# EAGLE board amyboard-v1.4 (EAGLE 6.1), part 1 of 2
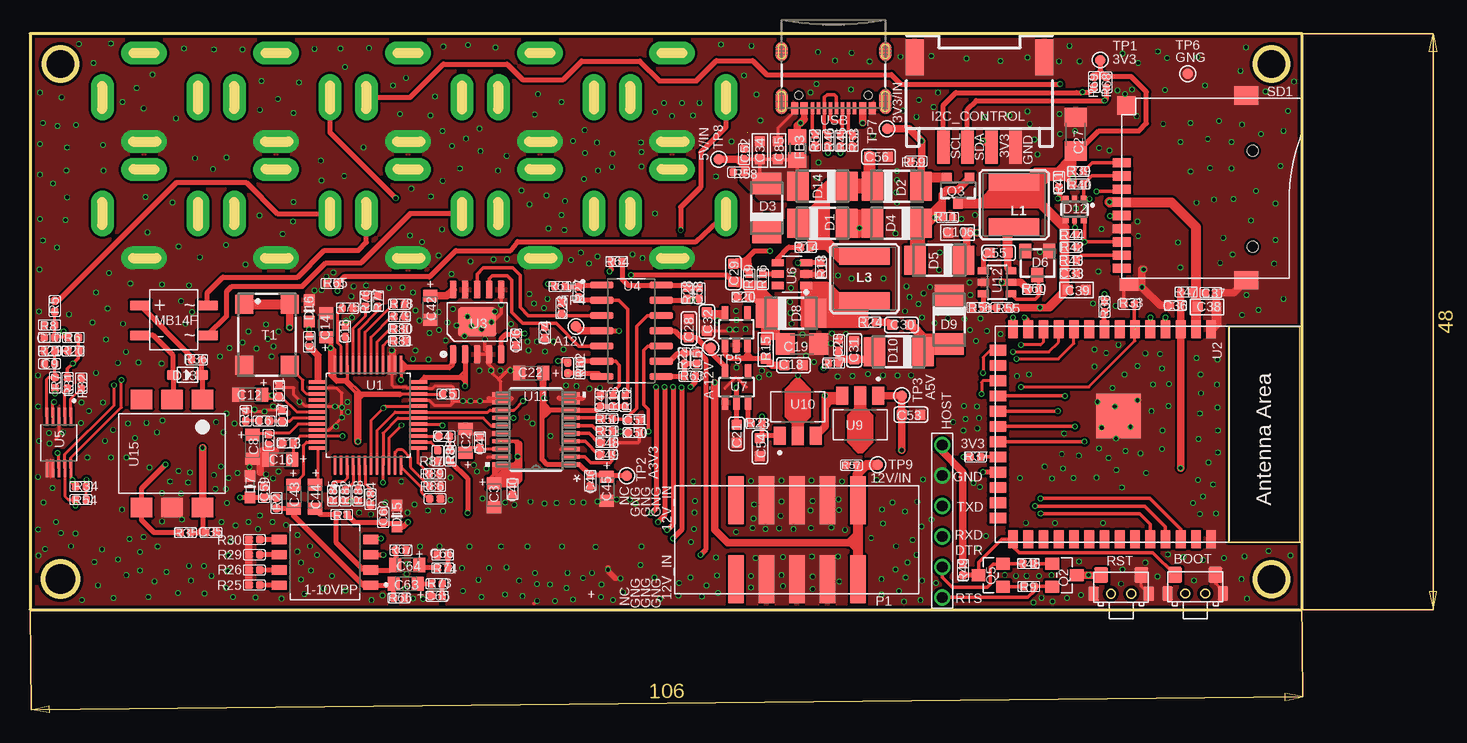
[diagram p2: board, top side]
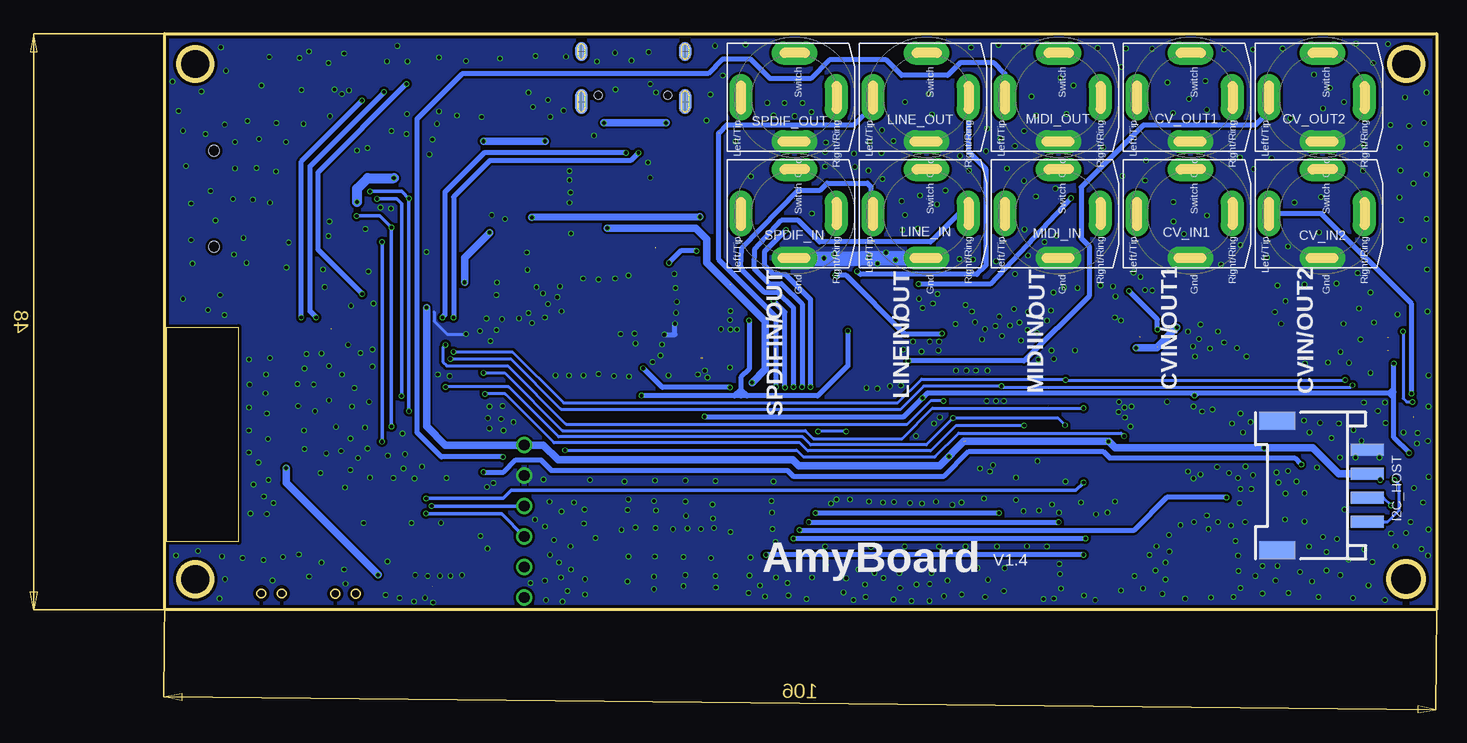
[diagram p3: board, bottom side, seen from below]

Size 117.22 x 56.61 mm. Coordinates in mm from the lower left corner, seen from the top.
Outline: 0,8.61 106,8.61 106,56.61 0,56.61 0,8.61
Outline: circle at 2.54,54.08 radius 1.37
Outline: circle at 2.54,11.15 radius 1.44
Outline: circle at 103.45,11.15 radius 1.37
Outline: circle at 103.45,54.08 radius 1.37
Copper layers (1*16): Top 0.035mm / dielectric 1.5mm / Bottom 0.035mm
Design rules: minimum track width 6mil, minimum drill 0.3mm, track to track 6mil, track to pad 6mil, pad to pad 6mil, via to via 6mil, smd to smd 0mil, copper to edge 10mil, drill to drill 8mil, minimum pad ring 3mil, minimum via ring 3mil, stop-mask expansion 0mil, vias tented up to drill 100mil, thermal gap 0mil
Net classes: 0 default: width 0.203 mm

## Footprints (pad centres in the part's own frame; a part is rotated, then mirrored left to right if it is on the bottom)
SW_218-4LPSTR = smd 1.27 x 0.76: 1 -3.81,1.905; 2 -3.81,0.635; 3 -3.81,-0.635; 4 -3.81,-1.905; 5 3.81,-1.905; 6 3.81,-0.635; 7 3.81,0.635; 8 3.81,1.905
2*4*3.5MM = smd 1.15 x 1.3: 1 -1.675,0; 2 1.675,0 | smd 0.9 x 1.2: 3 2.3,1.55; 4 -2.3,1.55
DISCRETE_C0402 = smd 0.635 x 0.635: 1 -0.445,0; 2 0.445,0
SMC_Z = smd 1 x 1.2: + -1,0; - 1,0
C0603 = smd 0.889 x 0.889: 1 0,0.762; 2 0,-0.762
C1206 = smd 1.6 x 1.8: 1 -1.4,0; 2 1.4,0
DISCRETE_C0603 = smd 0.889 x 0.889: 1 -0.762,0; 2 0.762,0
0603 = smd 0.889 x 0.889: 1 -0.762,0; 2 0.762,0
NV-PJ3410_SOCKET = drill 0.33 pad 1.93 long: GND 3.69,0; LEFT/TIP 0,-4.49; RIGHT/RING 0,3.459; SWITCH -3.674,0
DO-214AC = smd 1.8 x 2.4: A 2.025,0; C -2.025,0
TO236 = smd 1 x 1.2: A -1,-1; C 0,1; NC 1,-1
DIODE_PGB-0603MP = smd 0.95 x 0.9: 1 -0.889,0; 2 0.889,0
SOT363 = smd 0.5 x 0.5: 1 -0.75,-0.9; 3 0.75,-0.9; 4 0.75,0.9; 6 -0.75,0.9 | smd 0.4 x 0.5: 2 0,-0.9; 5 0,0.9
SOD323 = smd 1 x 0.8: + -1.2,0; - 1.2,0
R0805 = smd 1.3 x 1.5: 1 -0.95,0; 2 0.95,0
DEBUG*6 = drill 0.9: 1 0,0; 2 0,2.54; 3 0,5.08; 4 0,7.62; 5 0,10.16; 6 0,12.7
HW4-SMD-2.0-90D = smd 1.01 x 2.74: 1 -3,-0.1; 2 -1,-0.1; 3 1,-0.1; 4 3,-0.1 | smd 1.5 x 3: SS1 -5.4,7.4; SS2 5.4,7.4
CR54 = smd 4.2 x 1.4: P$1 0,1.85; P$2 0,-1.85
MBF = smd 1.676 x 0.813: AC1 2.8,1.2; AC2 2.8,-1.3; DCMINUS -2.8,-1.3; DCPLUS -2.8,1.2
2*5P-SMT2.54-HORN = smd 1.3 x 4: 1 -5.08,-3.3; 2 -2.54,-3.3; 3 0,-3.3; 4 2.54,-3.3; 5 5.08,-3.3; 6 5.08,3.3; 7 2.54,3.3; 8 0,3.3; 9 -2.54,3.3; 10 -5.08,3.3
PW20_TEX = smd 1.473 x 0.356: 1 -2.921,2.925; 2 -2.921,2.275; 3 -2.921,1.625; 4 -2.921,0.975; 5 -2.921,0.325; 6 -2.921,-0.325; 7 -2.921,-0.975; 8 -2.921,-1.625; 9 -2.921,-2.275; 10 -2.921,-2.925; 11 2.921,-2.925; 12 2.921,-2.275; 13 2.921,-1.625; 14 2.921,-0.975; 15 2.921,-0.325; 16 2.921,0.325; 17 2.921,0.975; 18 2.921,1.625; 19 2.921,2.275; 20 2.921,2.925
SOT23 = smd 1.016 x 1.143: 1 -0.95,-1.016; 2 0.95,-1.016; 3 0,1.016
SOT23-3 = smd 0.8 x 0.9: 1 -0.95,-1; 2 0.95,-1; 3 0,1.1
DISCRETE_R0402 = smd 0.635 x 0.635: 1 -0.445,0; 2 0.445,0
R0603 = smd 0.889 x 0.889: 1 -0.762,0; 2 0.762,0
9P-SMD-W/-RING = smd 1.524 x 0.762: 1 0,4.4; 2 0,3.3; 3 0,2.2; 4 0,1.1; 5 0,0; 6 0,-1.1; 7 0,-2.2; 8 0,-3.3; 9 0,-4.4 | smd 1.524 x 1.016: G1 0.6,-5.746 | smd 2.032 x 1.524: G2 10.373,-5.4; G3 10.373,10 | smd 1.524 x 1.524: G4 0.392,9.181 | hole 0.889: 10.9,-2.6; 10.9,5.4
SM77H = smd 1.6 x 1.5: 1 -2.55,-1.9; 2 2.55,-1.9; 3 2.55,1.9; 4 -2.55,1.9
TP_3535 = smd 0.889 x 0.889: T 0,0
QFP50P900X900X160-48N = smd 1.56 x 0.28: 1 -4.18,2.75; 2 -4.18,2.25; 3 -4.18,1.75; 4 -4.18,1.25; 5 -4.18,0.75; 6 -4.18,0.25; 7 -4.18,-0.25; 8 -4.18,-0.75; 9 -4.18,-1.25; 10 -4.18,-1.75; 11 -4.18,-2.25; 12 -4.18,-2.75; 25 4.18,-2.75; 26 4.18,-2.25; 27 4.18,-1.75; 28 4.18,-1.25; 29 4.18,-0.75; 30 4.18,-0.25; 31 4.18,0.25; 32 4.18,0.75; 33 4.18,1.25; 34 4.18,1.75; 35 4.18,2.25; 36 4.18,2.75 | smd 0.28 x 1.56: 13 -2.75,-4.18; 14 -2.25,-4.18; 15 -1.75,-4.18; 16 -1.25,-4.18; 17 -0.75,-4.18; 18 -0.25,-4.18; 19 0.25,-4.18; 20 0.75,-4.18; 21 1.25,-4.18; 22 1.75,-4.18; 23 2.25,-4.18; 24 2.75,-4.18; 37 2.75,4.18; 38 2.25,4.18; 39 1.75,4.18; 40 1.25,4.18; 41 0.75,4.18; 42 0.25,4.18; 43 -0.25,4.18; 44 -0.75,4.18; 45 -1.25,4.18; 46 -1.75,4.18; 47 -2.25,4.18; 48 -2.75,4.18
ESP32-­S2-­SOLO = smd 1.5 x 0.9: 1 -8.75,5.26; 2 -8.75,3.99; 3 -8.75,2.72; 4 -8.75,1.45; 5 -8.75,0.18; 6 -8.75,-1.09; 7 -8.75,-2.36; 8 -8.75,-3.63; 9 -8.75,-4.9; 10 -8.75,-6.17; 11 -8.75,-7.44; 12 -8.75,-8.71; 13 -8.75,-9.98; 14 -8.75,-11.25; 27 8.75,-11.25; 28 8.75,-9.98; 29 8.75,-8.71; 30 8.75,-7.44; 31 8.75,-6.17; 32 8.75,-4.9; 33 8.75,-3.63; 34 8.75,-2.36; 35 8.75,-1.09; 36 8.75,0.18; 37 8.75,1.45; 38 8.75,2.72; 39 8.75,3.99; 40 8.75,5.26 | smd 0.9 x 1.5: 15 -6.985,-12.5; 16 -5.715,-12.5; 17 -4.445,-12.5; 18 -3.175,-12.5; 19 -1.905,-12.5; 20 -0.635,-12.5; 21 0.635,-12.5; 22 1.905,-12.5; 23 3.175,-12.5; 24 4.445,-12.5; 25 5.715,-12.5; 26 6.985,-12.5 | smd 3.7 x 3.7: 41 -1.5,-2.46
ESOP-10-EP-150MIL = smd 1.5 x 0.6: 1 -2.7,2; 2 -2.7,1; 3 -2.7,0; 4 -2.7,-1; 5 -2.7,-2; 6 2.7,-2; 7 2.7,-1; 8 2.7,0; 9 2.7,1; 10 2.7,2 | smd 2.4 x 3.2: EP 0,0
SOIC127P600X175-14N = smd 1.97 x 0.6: 1 -2.475,3.81; 2 -2.475,2.54; 3 -2.475,1.27; 4 -2.475,0; 5 -2.475,-1.27; 6 -2.475,-2.54; 7 -2.475,-3.81; 8 2.475,-3.81; 9 2.475,-2.54; 10 2.475,-1.27; 11 2.475,0; 12 2.475,1.27; 13 2.475,2.54; 14 2.475,3.81
SOP50P490X110-10N = smd 1.47 x 0.28: 1 -2.15,1; 2 -2.15,0.5; 3 -2.15,0; 4 -2.15,-0.5; 5 -2.15,-1; 6 2.15,-1; 7 2.15,-0.5; 8 2.15,0; 9 2.15,0.5; 10 2.15,1
SOT-23-6 = smd 1 x 0.6: 1 -1.2,0.95; 2 -1.2,0; 3 -1.2,-0.95; 4 1.2,-0.95; 5 1.2,0; 6 1.2,0.95
SOT25 = smd 0.55 x 1.2: 1 -0.95,-1.3; 2 0,-1.3; 3 0.95,-1.3; 4 0.95,1.3; 5 -0.95,1.3
VREG_UA78L05ACPKG4 = smd 1.5 x 1: 1 -2,1.5; 2 -2,0; 3 -2,-1.5
SOT23-6 = smd 0.6 x 0.9: 1 -0.95,-1.15; 2 0,-1.15; 3 0.95,-1.15; 4 0.95,1.15; 5 0,1.15; 6 -0.95,1.15
SOP-6-2.54MM = smd 1.6 x 1.8: 1 -4.5,2.54; 2 -4.5,0; 3 -4.5,-2.54; 4 4.5,-2.54; 5 4.5,0; 6 4.5,2.54
USB-C-16P-5 = smd 0.3 x 1: A5 -1.25,-0.34; A6 -0.25,-0.34; A7 0.25,-0.34; A8 1.25,-0.34; B5 1.75,-0.34; B6 0.75,-0.34; B7 -0.75,-0.34; B8 -1.75,-0.34 | smd 0.6 x 1: GND -3.225,-0.34; GND2 3.225,-0.34; VBUS1 -2.45,-0.34; VBUS2 2.45,-0.34 | smd 1 x 2.1: SHLD1 -4.32,-0.915; SHLD2 4.32,-0.915 | smd 1 x 2.1 bottom: SHLD3 -4.32,-0.915; SHLD4 4.32,-0.915 | smd 1 x 1.6: SHLD5 -4.32,-5.095; SHLD8 4.32,-5.095 | smd 1 x 1.6 bottom: SHLD6 -4.32,-5.095; SHLD7 4.32,-5.095 | hole 0.65: -2.89,-1.445; 2.89,-1.445

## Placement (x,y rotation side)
1-10VPP  218-4LPSTR  [SW_218-4LPSTR]  24.59,12.55 180 top
BOOT  TS24CA  [2*4*3.5MM]  97.1,11.51 180 top
C1  100nF  [DISCRETE_C0402]  23.27,30.94 90 top
C2  10uF/10V/TAN  [SMC_Z]  36.28,22.68 90 top
C3  10uF/10V/TAN  [SMC_Z]  38.66,18.16 270 top
C4  100nF  [DISCRETE_C0402]  34.52,23.06 0 top
C5  100nF  [DISCRETE_C0402]  34.82,26.57 0 top
C6  68nF  [DISCRETE_C0402]  19.51,24.33 0 top
C7  100nF  [DISCRETE_C0402]  19.86,22.76 270 top
C8  10uF/10V/TAN  [SMC_Z]  18.54,22.2 270 top
C9  1nF  [DISCRETE_C0402]  1.63,29.11 180 top
C10  1nF  [DISCRETE_C0402]  1.63,31.29 180 top
C11  100nF  [DISCRETE_C0402]  20.75,26.85 90 top
C12  10uF/10V/TAN  [SMC_Z]  18.36,26.52 180 top
C13  100nF  [DISCRETE_C0402]  21.51,22.51 180 top
C14  10uF/10V/TAN  [SMC_Z]  24.69,32.31 90 top
C15  100nF  [DISCRETE_C0402]  26.26,31.8 90 top
C16  10uF/10V/TAN  [SMC_Z]  20.85,21.11 180 top
C17  4.7nF  [DISCRETE_C0402]  21.01,24.77 270 top
C18  10uF  [C0603]  63.63,28.98 90 top
C19  22uF  [C1206]  64.34,30.74 0 top
C20  100nF  [DISCRETE_C0402]  59.41,34.67 0 top
C21  1uF  [C0603]  58.88,23.27 180 top
C22  10uF/10V/TAN  [SMC_Z]  41.78,28.32 180 top
C23  100nF  [DISCRETE_C0402]  44.3,33.73 270 top
C24  100nF  [DISCRETE_C0402]  42.9,31.7 90 top
C25  100nF  [DISCRETE_C0402]  67.41,30.66 90 top
C26  100nF  [DISCRETE_C0402]  40.51,31.12 90 top
C27  22uF  [C1206]  87.15,48.24 90 top
C28  1uF  [C0603]  54.91,32.06 180 top
C29  22pF  [C0603]  58.62,36.68 180 top
C30  1uF  [C0603]  72.62,32.34 90 top
C31  10uF  [C0603]  68.68,30.23 0 top
C32  1uF  [C0603]  56.41,32.61 0 top
C33  100nF  [DISCRETE_C0402]  86.74,36.63 180 top
C34  10uF  [DISCRETE_C0603]  60.83,46.89 270 top
C35  100nF  [DISCRETE_C0402]  15.09,15.04 0 top
C36  100nF  [DISCRETE_C0402]  95.45,33.96 0 top
C37  100nF  [DISCRETE_C0402]  98.4,35.03 180 top
C38  10uF  [DISCRETE_C0603]  98.09,33.83 0 top
C39  10uF  [DISCRETE_C0603]  87.22,35.26 180 top
C40  100nF  [DISCRETE_C0402]  40.21,18.64 270 top
C41  100nF  [DISCRETE_C0402]  37.49,22.56 270 top
C42  10uF/10V/TAN  [SMC_Z]  33.35,33.76 270 top
C43  10uF/10V/TAN  [SMC_Z]  21.97,18.04 270 top
C44  10uF/10V/TAN  [SMC_Z]  23.75,18.01 270 top
C45  10uF/10V/TAN  [SMC_Z]  48.06,18.67 270 top
C46  100nF  [DISCRETE_C0402]  46.69,19.36 270 top
C47  100nF  [DISCRETE_C0402]  47.55,26.01 90 top
C48  2.2uF  [DISCRETE_C0402]  48.06,22.53 180 top
C49  2.2uF  [DISCRETE_C0402]  48.03,21.54 180 top
C50  2.2nF  [DISCRETE_C0402]  50.34,23.37 180 top
C51  2.2nF  [DISCRETE_C0402]  50.34,24.46 180 top
C52  100nF  [DISCRETE_C0402]  59.51,46.58 270 top
C53  1uF  [C0603]  73.41,24.87 90 top
C54  1uF  [C0603]  60.83,22.15 0 top
C55  22nF  [C0603]  80.72,38.36 90 top
C56  10uF  [C0603]  70.71,46.36 90 top
C57  220pF  [DISCRETE_C0402]  55.55,29.54 270 top
C58  220pF  [DISCRETE_C0402]  55.78,34.98 90 top
C59  100pF  [DISCRETE_C0402]  19.51,18.39 270 top
C60  100pF  [DISCRETE_C0402]  29.44,16.31 270 top
C63  10uF/10V/TAN  [SMC_Z]  31.32,10.77 180 top
C64  10uF/10V/TAN  [SMC_Z]  31.45,12.35 180 top
C65  10nF  [DISCRETE_C0402]  33.91,9.73 0 top
C66  10nF  [DISCRETE_C0402]  34.39,13.16 0 top
C85  10uF  [DISCRETE_C0603]  62.33,46.89 270 top
C106  22uF/16V  [0603]  77.29,40.03 180 top
CV_IN1  NV-PJ3410_STEREO  [NV-PJ3410_SOCKET]  20.5,41.61 270 bottom
CV_IN2  NV-PJ3410_STEREO  [NV-PJ3410_SOCKET]  9.5,41.61 270 bottom
CV_OUT1  NV-PJ3410_STEREO  [NV-PJ3410_SOCKET]  20.5,51.31 270 bottom
CV_OUT2  NV-PJ3410_STEREO  [NV-PJ3410_SOCKET]  9.5,51.31 270 bottom
D1  SS34  [DO-214AC]  66.04,40.82 0 top
D2  SS34  [DO-214AC]  72.24,43.89 0 top
D3  SS34  [DO-214AC]  61.39,42.09 90 top
D4  SS34  [DO-214AC]  72.24,40.82 180 top
D5  SS34  [DO-214AC]  75.77,37.72 180 top
D6  BZX84C3V3  [TO236]  83.95,37.49 180 top
D7  DIODE_PGB-0603MP  [DIODE_PGB-0603MP]  18.34,18.85 270 top
D8  SS34  [DO-214AC]  63.42,33.3 0 top
D9  SS34  [DO-214AC]  76.61,32.77 270 top
D10  SS34  [DO-214AC]  72.39,30.1 180 top
D12  SMF05C  [SOT363]  87.05,41.96 180 top
D13  1N4148WS  [SOD323]  13.13,28.17 0 top
D14  SS34  [DO-214AC]  66.04,43.89 180 top
D15  DIODE_PGB-0603MP  [DIODE_PGB-0603MP]  30.58,16.41 270 top
D16  DIODE_PGB-0603MP  [DIODE_PGB-0603MP]  23.27,33.53 270 top
FB3  100Mhz@120R  [R0805]  63.96,47.04 270 top
HOST  DEBUG6  [DEBUG*6]  76.02,22.33 180 top
I2C_CONTROL  HW4-SMD-2.0  [HW4-SMD-2.0-90D]  79.12,47.25 0 top
I2C_HOST  HW4-SMD-2.0  [HW4-SMD-2.0-90D]  5.89,18.95 90 bottom
L1  10µH  [CR54]  82.02,42.37 180 top
L3  3.3µH/±30%/3.4A  [CR54]  69.55,36.2 0 top
LINE_IN  NV-PJ3410_STEREO  [NV-PJ3410_SOCKET]  42.5,41.61 270 bottom
LINE_OUT  NV-PJ3410_STEREO  [NV-PJ3410_SOCKET]  42.5,51.31 270 bottom
MB14F  MB14F  [MBF]  11.99,32.77 0 top
MIDI_IN  NV-PJ3410_STEREO  [NV-PJ3410_SOCKET]  31.5,41.61 270 bottom
MIDI_OUT  NV-PJ3410_STEREO  [NV-PJ3410_SOCKET]  31.5,51.31 270 bottom
P1  2X5P-SMT2.542  [2*5P-SMT2.54-HORN]  63.91,14.43 0 top
PCM5101  U11  [PW20_TEX]  42.16,23.62 180 top
Q2  S8050  [SOT23]  86.21,11.48 270 top
Q3  DMP4065SQ  [SOT23-3]  77.34,43.59 180 top
Q5  S8050  [SOT23]  80.06,11.48 90 top
R1  5.1K  [DISCRETE_R0402]  25.98,16.54 0 top
R2  5.1K  [DISCRETE_R0402]  20.55,17.5 90 top
R3  150R  [DISCRETE_R0402]  35.03,21.44 270 top
R4  680R  [DISCRETE_R0402]  17.98,24.77 90 top
R5  39.7K  [DISCRETE_R0402]  2.06,33.91 90 top
R6  13.1K  [DISCRETE_R0402]  3.61,31.29 0 top
R7  39.7K  [DISCRETE_R0402]  2.08,27.53 270 top
R8  10K  [DISCRETE_R0402]  1.63,32.34 0 top
R9  10K  [DISCRETE_R0402]  83.24,10.54 0 top
R10  30K  [DISCRETE_R0402]  45.8,28.75 90 top
R11  100K  [DISCRETE_R0402]  76.45,41.3 180 top
R12  10K  [DISCRETE_R0402]  49.61,26.01 270 top
R13  10K  [DISCRETE_R0402]  48.59,26.01 270 top
R14  10K  [DISCRETE_R0402]  64.64,38.81 180 top
R15  10R  [R0603]  61.32,30.3 90 top
R16  0R  [DISCRETE_R0402]  61.06,36.15 90 top
R17  10R  [DISCRETE_R0402]  66.98,29.16 0 top
R18  4.65K  [DISCRETE_R0402]  65.91,37.09 270 top
R19  100K  [DISCRETE_R0402]  59.94,36.15 90 top
R20  13.1K  [DISCRETE_R0402]  3.61,30.18 0 top
R21  10K  [DISCRETE_R0402]  1.63,30.18 0 top
R22  51K  [DISCRETE_R0402]  54.53,29.54 90 top
R23  1K  [DISCRETE_R0402]  60.55,24.13 180 top
R24  2R  [DISCRETE_R0402]  70,32.56 180 top
R25  2.2K  [DISCRETE_R0402]  18.69,10.67 0 top
R26  2.2K  [DISCRETE_R0402]  18.69,11.91 0 top
R27  30K  [DISCRETE_R0402]  45.72,35.08 270 top
R28  51K  [DISCRETE_R0402]  54.74,34.98 270 top
R29  22K  [DISCRETE_R0402]  18.69,13.18 0 top
R30  22K  [DISCRETE_R0402]  18.69,14.45 0 top
R31  10K  [DISCRETE_R0402]  3.12,27.51 270 top
R32  10K  [DISCRETE_R0402]  4.27,27.48 270 top
R33  10K  [DISCRETE_R0402]  91.59,34.06 0 top
R34  5.1K  [DISCRETE_R0402]  4.24,18.87 180 top
R35  470R  [DISCRETE_R0402]  12.95,15.04 180 top
R36  220R  [DISCRETE_R0402]  13.89,29.44 0 top
R37  22R  [DISCRETE_R0402]  78.79,21.34 0 top
R38  22R  [DISCRETE_R0402]  89.53,33.83 270 top
R39  10K  [DISCRETE_R0402]  87.35,45.14 180 top
R40  10K  [DISCRETE_R0402]  87.35,44.07 180 top
R41  10K  [DISCRETE_R0402]  85.75,44.25 90 top
R42  10K  [DISCRETE_R0402]  86.74,38.81 180 top
R43  10K  [DISCRETE_R0402]  86.74,37.72 180 top
R44  NC  [DISCRETE_R0402]  86.74,39.88 180 top
R45  51R  [DISCRETE_R0402]  67.54,47.68 270 top
R46  51R  [DISCRETE_R0402]  66.5,47.7 270 top
R47  10K  [DISCRETE_R0402]  96.34,35.08 0 top
R48  10K  [DISCRETE_R0402]  83.19,12.45 180 top
R49  10K  [DISCRETE_R0402]  77.75,11.94 90 top
R50  470R  [DISCRETE_R0402]  48.08,24.54 180 top
R51  470R  [DISCRETE_R0402]  48.08,23.5 180 top
R52  5.1K  [DISCRETE_R0402]  65.43,47.73 270 top
R53  5.1K  [DISCRETE_R0402]  68.55,47.65 270 top
R54  5.1K  [DISCRETE_R0402]  4.24,17.78 180 top
R55  100K  [DISCRETE_R0402]  81,33.78 180 top
R56  22.2K  [DISCRETE_R0402]  78.99,33.78 180 top
R57  100K  [DISCRETE_R0402]  68.45,20.65 180 top
R58  100K  [DISCRETE_R0402]  59.05,45.06 180 top
R59  100K  [DISCRETE_R0402]  73.84,45.98 180 top
R60  100K  [DISCRETE_R0402]  83.62,35.28 0 top
R61  100R  [DISCRETE_R0402]  44.17,35.54 0 top
R62  100R  [DISCRETE_R0402]  44.81,28.75 270 top
R63  100R  [DISCRETE_R0402]  54.99,28.07 180 top
R64  100R  [DISCRETE_R0402]  48.9,37.62 0 top
R65  75R  [DISCRETE_R0402]  25.17,35.79 180 top
R66  51K  [DISCRETE_R0402]  30.76,9.58 0 top
R67  51K  [DISCRETE_R0402]  30.91,13.56 0 top
R68  5.1K  [DISCRETE_R0402]  89.69,52.55 90 top
R69  5.1K  [DISCRETE_R0402]  88.67,52.58 90 top
R73  100  [DISCRETE_R0402]  33.91,10.77 180 top
R74  100  [DISCRETE_R0402]  34.39,12.09 180 top
R75  10K  [DISCRETE_R0402]  26.47,33.73 0 top
R76  10K  [DISCRETE_R0402]  27.97,34.32 90 top
R77  10K  [DISCRETE_R0402]  28.98,34.32 90 top
R78  10K  [DISCRETE_R0402]  30.78,34.06 0 top
R79  10K  [DISCRETE_R0402]  30.78,33.05 0 top
R80  10K  [DISCRETE_R0402]  30.78,32.03 0 top
R81  10K  [DISCRETE_R0402]  30.78,31.01 0 top
R82  10K  [DISCRETE_R0402]  26.29,18.11 270 top
R83  10K  [DISCRETE_R0402]  27.36,18.11 270 top
R84  10K  [DISCRETE_R0402]  28.37,17.81 270 top
R85  10K  [DISCRETE_R0402]  25.27,18.11 270 top
R86  10K  [DISCRETE_R0402]  33.76,17.86 0 top
R87  10K  [DISCRETE_R0402]  33.71,19.94 0 top
R88  10K  [DISCRETE_R0402]  33.99,21.44 270 top
R89  10K  [DISCRETE_R0402]  33.73,18.9 0 top
RST  TS24CA  [2*4*3.5MM]  90.93,11.49 180 top
SD1  SD  [9P-SMD-W/-RING]  90.98,41.45 0 top
SPDIF_IN  NV-PJ3410_STEREO  [NV-PJ3410_SOCKET]  53.5,41.61 270 bottom
SPDIF_OUT  NV-PJ3410_STEREO  [NV-PJ3410_SOCKET]  53.5,51.31 270 bottom
T1  SM77H  [SM77H]  19.74,31.52 270 top
TP1  [TP_3535]  89.18,54.41 0 top
TP2  [TP_3535]  49.73,19.76 90 top
TP3  [TP_3535]  72.64,26.44 90 top
TP4  [TP_3535]  45.49,32.21 90 top
TP5  [TP_3535]  56.72,30.46 90 top
TP6  [TP_3535]  96.47,53.26 90 top
TP7  [TP_3535]  71.42,48.69 0 top
TP8  [TP_3535]  57.4,46.15 0 top
TP9  [TP_3535]  70.64,20.68 0 top
U1  PCM9211PT  [QFP50P900X900X160-48N]  28.17,24.82 90 top
U2  ESP32­S2­SOLO  [ESP32-­S2-­SOLO]  93.17,23.24 270 top
U3  GP8413  [ESOP-10-EP-150MIL]  37.26,32.59 90 top
U4  TL074CD  [SOIC127P600X175-14N]  50.11,31.85 0 top
U5  ADS1015IDGSR  [SOP50P490X110-10N]  2.41,22.53 270 top
U6  HX3608  [SOT-23-6]  63.5,36.58 180 top
U7  TS5205  [SOT25]  58.88,27.15 0 top
U8  TS5205  [SOT25]  58.85,31.98 0 top
U9  78L05-150  [VREG_UA78L05ACPKG4]  69.19,24.44 270 top
U10  78L33  [VREG_UA78L05ACPKG4]  63.98,25.1 90 top
U12  MT2492  [SOT23-6]  80.59,35.89 270 top
U15  H11L1SR2M  [SOP-6-2.54MM]  11.84,21.62 270 top
USB  USB-C  [USB-C-16P-5]  66.95,50.04 180 top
